FUNCTION FC 95 : VOID
TITLE =BLOCK FOR MAIN MOTOR
AUTHOR : Esposito
FAMILY : EGAL_srl
NAME : MAIN_MOT
VERSION : 0.1


VAR_TEMP
  L_speed : REAL ;
  L_speed_up : REAL ;
  L_speed_dw : REAL ;
END_VAR
BEGIN
NETWORK
TITLE =CONDITION FOR MAIN MOTOR
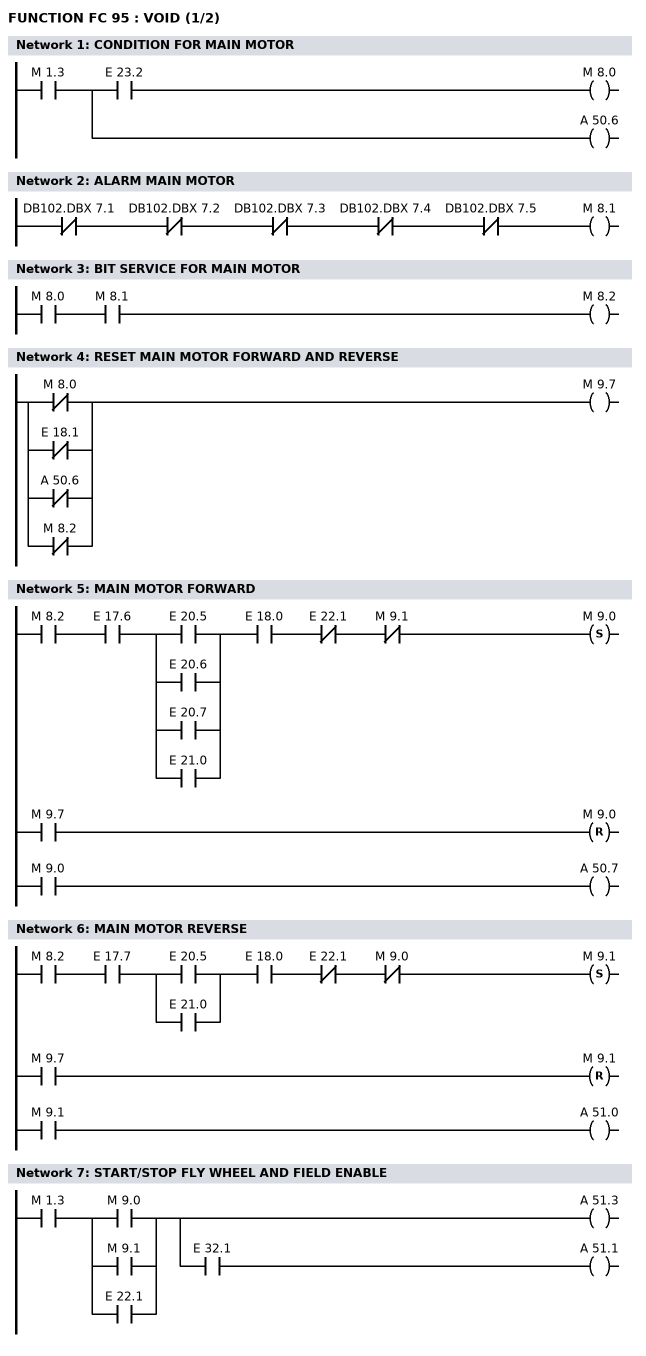
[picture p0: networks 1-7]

      U     M      1.3;
      =     L     12.0;
      U     L     12.0;
      U     E     23.2;
      =     M      8.0;
      U     L     12.0;
      BLD   102;
      =     A     50.6;
NETWORK
TITLE =ALARM MAIN MOTOR

      UN    DB102.DBX    7.1;
      UN    DB102.DBX    7.2;
      UN    DB102.DBX    7.3;
      UN    DB102.DBX    7.4;
      UN    DB102.DBX    7.5;
      =     M      8.1;
NETWORK
TITLE =BIT SERVICE FOR MAIN MOTOR

      U     M      8.0;
      U     M      8.1;
      =     M      8.2;
NETWORK
TITLE =RESET MAIN MOTOR FORWARD AND REVERSE

      ON    M      8.0;
      ON    E     18.1;
      ON    A     50.6;
      ON    M      8.2;
      =     M      9.7;
NETWORK
TITLE =MAIN MOTOR FORWARD

      U     M      8.2;
      U     E     17.6;
      U(    ;
      O     E     20.5;
      O     E     20.6;
      O     E     20.7;
      O     E     21.0;
      )     ;
      U     E     18.0;
      UN    E     22.1;
      UN    M      9.1;
      S     M      9.0;
      U     M      9.7;
      R     M      9.0;
      U     M      9.0;
      =     A     50.7;
NETWORK
TITLE =MAIN MOTOR REVERSE

      U     M      8.2;
      U     E     17.7;
      U(    ;
      O     E     20.5;
      O     E     21.0;
      )     ;
      U     E     18.0;
      UN    E     22.1;
      UN    M      9.0;
      S     M      9.1;
      U     M      9.7;
      R     M      9.1;
      U     M      9.1;
      =     A     51.0;
NETWORK
TITLE =START/STOP FLY WHEEL AND FIELD ENABLE

      U     M      1.3;
      U(    ;
      O     M      9.0;
      O     M      9.1;
      O     E     22.1;
      )     ;
      =     L     12.0;
      U     L     12.0;
      BLD   102;
      =     A     51.3;
      U     L     12.0;
      U     E     32.1;
      =     A     51.1;
NETWORK
TITLE =ENABLE MAIN MOTOR
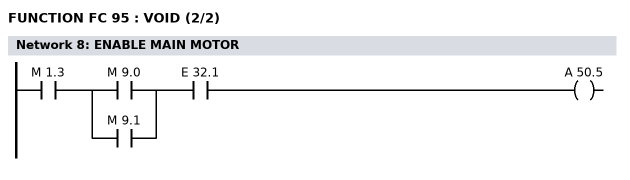
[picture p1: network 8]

      U     M      1.3;
      U(    ;
      O     M      9.0;
      O     M      9.1;
      )     ;
      U     E     32.1;
      =     A     50.5;
NETWORK
TITLE =MINIMAL AND MAXIMAL VALUE IN MODE DIE CHANGE

      U     M      1.0;
      U     E     21.0;
      =     L     12.0;
      U(    ;
      U     L     12.0;
      SPBNB _001;
      L     1.600000e+001;
      T     DB15.DBD  236;
      SET   ;
      SAVE  ;
      CLR   ;
_001: U     BIE;
      )     ;
      SPBNB _002;
      L     1.600000e+001;
      T     DB15.DBD  240;
_002: NOP   0;
      U     L     12.0;
      SPBNB _003;
      L     5;
      T     DB15.DBW  244;
_003: NOP   0;
NETWORK
TITLE =MINIMAL AND MAXIMAL VALUE IN MODE INCHING

      U     M      1.0;
      U     E     20.5;
      =     L     12.0;
      U(    ;
      U     L     12.0;
      SPBNB _004;
      L     1.600000e+001;
      T     DB15.DBD  236;
      SET   ;
      SAVE  ;
      CLR   ;
_004: U     BIE;
      )     ;
      SPBNB _007;
      L     1.600000e+001;
      T     DB15.DBD  240;
_007: NOP   0;
      U     L     12.0;
      SPBNB _00f;
      L     4;
      T     DB15.DBW  244;
_00f: NOP   0;
NETWORK
TITLE =MINIMAL AND MAXIMAL VALUE IN MODE SINGLE STROKE MANUAL

      U     M      1.0;
      U     E     21.1;
      =     L     12.0;
      U(    ;
      U     L     12.0;
      SPBNB _013;
      L     1.600000e+001;
      T     DB15.DBD  236;
      SET   ;
      SAVE  ;
      CLR   ;
_013: U     BIE;
      )     ;
      SPBNB _014;
      L     1.600000e+001;
      T     DB15.DBD  240;
_014: NOP   0;
      U     L     12.0;
      SPBNB _017;
      L     3;
      T     DB15.DBW  244;
_017: NOP   0;
NETWORK
TITLE =MINIMAL AND MAXIMAL VALUE IN MODE SINGLE STROKE AUTOMATIC

      U     M      1.0;
      U     E     20.6;
      =     L     12.0;
      U(    ;
      U     L     12.0;
      SPBNB _020;
      L     1.600000e+001;
      T     DB15.DBD  236;
      SET   ;
      SAVE  ;
      CLR   ;
_020: U     BIE;
      )     ;
      SPBNB _023;
      L     1.600000e+001;
      T     DB15.DBD  240;
_023: NOP   0;
      U     L     12.0;
      SPBNB _026;
      L     2;
      T     DB15.DBW  244;
_026: NOP   0;
NETWORK
TITLE =MINIMAL AND MAXIMAL VALUE IN MODE CONTINOUS

      U     M      1.0;
      U     E     20.7;
      =     L     12.0;
      U(    ;
      U     L     12.0;
      SPBNB _02e;
      L     1.600000e+001;
      T     DB15.DBD  236;
      SET   ;
      SAVE  ;
      CLR   ;
_02e: U     BIE;
      )     ;
      SPBNB _033;
      L     4.000000e+001;
      T     DB15.DBD  240;
_033: NOP   0;
      U     L     12.0;
      SPBNB _037;
      L     1;
      T     DB15.DBW  244;
_037: NOP   0;
      U     L     12.0;
      BLD   102;
      =     M     17.7;
NETWORK
TITLE =SET VALUE MINIMAL SPEED MAIN MOTOR
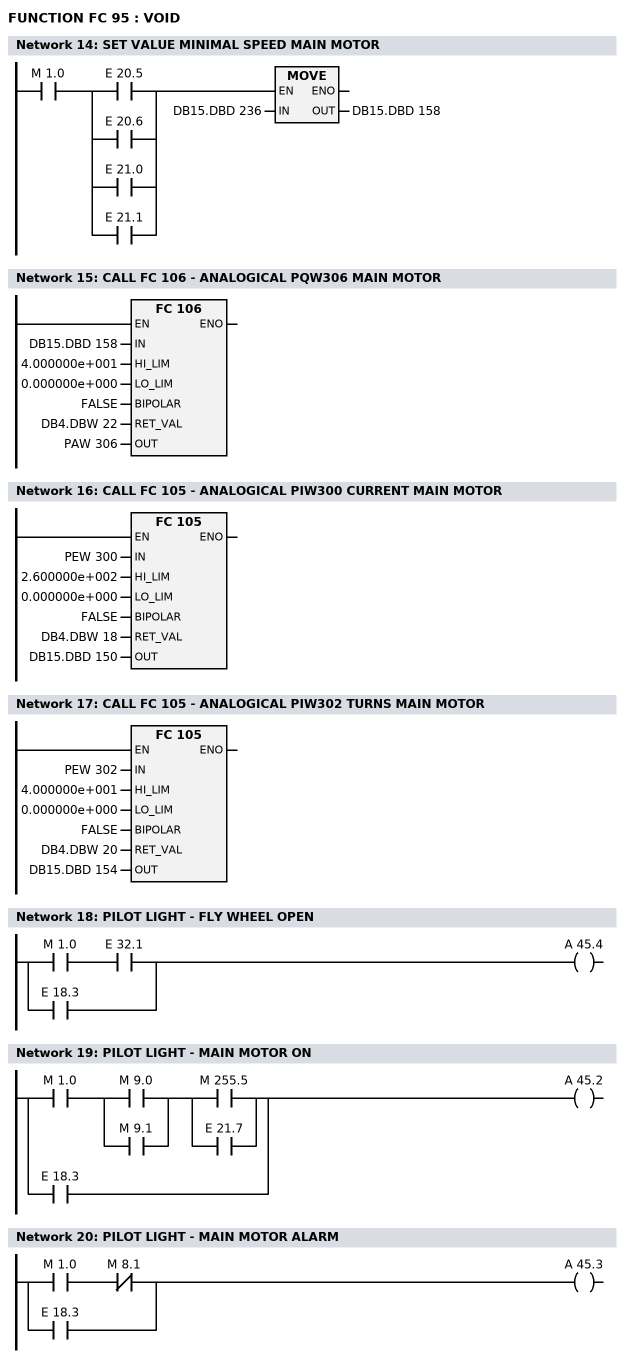
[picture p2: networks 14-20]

      U     M      1.0;
      U(    ;
      O     E     20.5;
      O     E     20.6;
      O     E     21.0;
      O     E     21.1;
      )     ;
      SPBNB _03b;
      L     DB15.DBD  236;
      T     DB15.DBD  158;
_03b: NOP   0;
NETWORK
TITLE =CALL FC 106 - ANALOGICAL PQW306 MAIN MOTOR

      CALL FC   106 (
           IN                       := DB15.DBD  158,
           HI_LIM                   := 4.000000e+001,
           LO_LIM                   := 0.000000e+000,
           BIPOLAR                  := FALSE,
           RET_VAL                  := DB4.DBW   22,
           OUT                      := PAW  306);

NETWORK
TITLE =CALL FC 105 - ANALOGICAL PIW300 CURRENT MAIN MOTOR

      CALL FC   105 (
           IN                       := PEW  300,
           HI_LIM                   := 2.600000e+002,
           LO_LIM                   := 0.000000e+000,
           BIPOLAR                  := FALSE,
           RET_VAL                  := DB4.DBW   18,
           OUT                      := DB15.DBD  150);

NETWORK
TITLE =CALL FC 105 - ANALOGICAL PIW302 TURNS MAIN MOTOR

      CALL FC   105 (
           IN                       := PEW  302,
           HI_LIM                   := 4.000000e+001,
           LO_LIM                   := 0.000000e+000,
           BIPOLAR                  := FALSE,
           RET_VAL                  := DB4.DBW   20,
           OUT                      := DB15.DBD  154);

NETWORK
TITLE =PILOT LIGHT - FLY WHEEL OPEN

      U     M      1.0;
      U     E     32.1;
      O     E     18.3;
      =     A     45.4;
NETWORK
TITLE =PILOT LIGHT - MAIN MOTOR ON

      U     M      1.0;
      U(    ;
      O     M      9.0;
      O     M      9.1;
      )     ;
      U(    ;
      O     M    255.5;
      O     E     21.7;
      )     ;
      O     E     18.3;
      =     A     45.2;
NETWORK
TITLE =PILOT LIGHT - MAIN MOTOR ALARM

      U     M      1.0;
      UN    M      8.1;
      O     E     18.3;
      =     A     45.3;
END_FUNCTION

